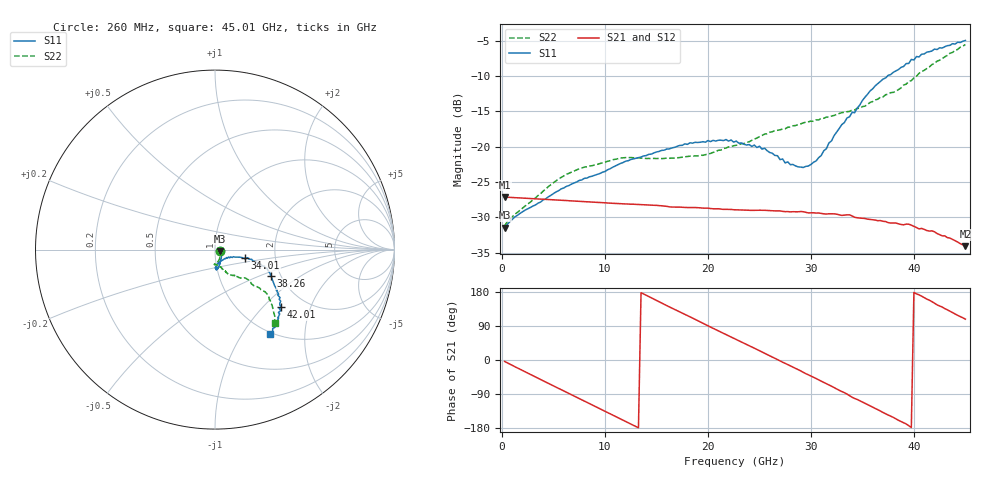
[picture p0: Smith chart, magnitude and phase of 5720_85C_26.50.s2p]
! Device:  ADRF5720
! Description: 0.5dB LSB GaAs MMIC 6-bit Digital Attenuator
! Frequency:  0.000009 -  40 GHz
! Ports:
!	RF1	= Port 1
!	RF2	= Port 2
! Vdd:  3.3 Volt
! Vss:  -3.3 Volt
! Control:  0/3.3 Volt
! State:  26.50 dB attenuation
! Data:  The device was measured using G-S-G Probes on a matrix board.
!  Data was collected using an calibrated 4 port network analyzer.
!  The reference plane for this measurement is at the launchers.
! Note:  Analog Devices supplies this data as a sample of measured data
!  for this product.  Your particular data for this product may vary.
!  Data was taken at 85 degrees C.
!  Analog Devices reserves the right to change this data at anytime.
# GHZ S DB R 45.0
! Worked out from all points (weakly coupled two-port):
!   180 points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, 260 MHz to 45.01 GHz, reference 45 ohm
!   highest |S21| = -27.13 dB at 260 MHz (marker M1); lowest = -34.1 dB at 45.01 GHz (marker M2)
!   lowest |S11| = -31.5 dB at 260 MHz (marker M3), VSWR 1.05, Z = 47.3 - j0.763 ohm
!   |S11| at or under -10 dB: start of sweep to 37.46 GHz
!   |S22| runs from -31.2 to -5.6 dB; largest |S21 - S12| = 0.00029
!   S11 on the Smith chart (normalised r, x): 260 MHz: 1.05, -0.02; 34.01 GHz: 1.40, -0.14; 38.26 GHz: 1.77, -0.59; 42.01 GHz: 1.52, -1.28; 45.01 GHz: 0.97, -1.34
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0.26  -31.46 -17.5  -27.13 -3.8  -27.12 -3.8  -31.19 -17.8
1.26  -29.93 -3.4  -27.22 -17.7  -27.21 -17.6  -29.56 -12.0
5.01  -26.63 -39.1  -27.51 -68.3  -27.50 -68.3  -25.08 -61.8
7.76  -24.70 -53.4  -27.75 -105.1  -27.74 -105.1  -23.02 -78.2
11.51  -22.38 -67.5  -28.06 -155.3  -28.05 -155.2  -21.62 -91.6
15.26  -20.68 -75.5  -28.34 153.7  -28.32 153.9  -21.67 -92.8
18.26  -19.46 -81.1  -28.61 114.0  -28.59 114.2  -21.35 -86.5
22.76  -19.21 -86.7  -28.93 54.0  -28.91 54.2  -19.81 -72.8
25.51  -20.22 -85.4  -29.00 17.8  -28.99 18.1  -18.23 -68.4
27.51  -22.30 -78.3  -29.19 -8.9  -29.17 -8.6  -17.47 -63.8
28.76  -22.86 -61.6  -29.21 -25.1  -29.19 -24.8  -16.88 -63.8
30.26  -22.21 -41.2  -29.35 -45.5  -29.34 -45.3  -16.43 -62.0
31.01  -21.25 -28.5  -29.44 -55.9  -29.42 -55.7  -15.99 -60.5
34.01  -15.15 -16.0  -29.80 -98.3  -29.78 -98.0  -14.82 -53.5
34.26  -15.20 -17.4  -29.99 -101.6  -29.98 -101.3  -14.82 -52.5
36.26  -11.40 -17.7  -30.38 -128.0  -30.36 -127.8  -13.40 -48.0
37.76  -9.81 -22.1  -30.80 -148.4  -30.79 -148.1  -12.37 -42.9
38.26  -9.30 -25.2  -30.80 -155.3  -30.78 -155.0  -12.18 -42.4
39.76  -7.67 -33.0  -31.10 -178.0  -31.07 -177.7  -10.66 -43.1
42.01  -6.21 -41.0  -32.04 149.9  -32.00 150.1  -8.24 -40.9
43.51  -5.68 -47.0  -32.93 128.7  -32.90 129.2  -6.80 -45.3
45.01  -4.99 -57.0  -34.07 107.8  -34.02 107.9  -5.57 -50.6
